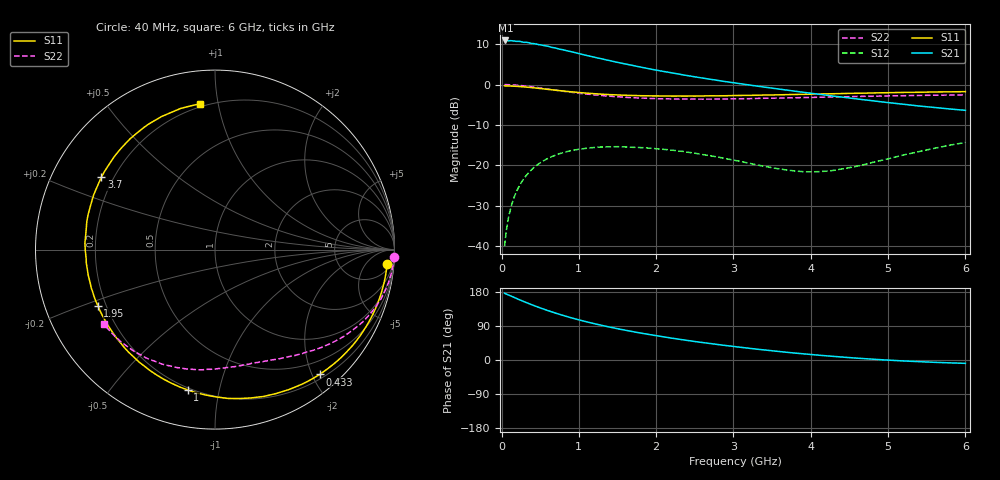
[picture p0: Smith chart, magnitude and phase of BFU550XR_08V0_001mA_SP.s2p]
! Filename:  P:\Prog\Test\Noise\ATS_data\Testdata_Net\03 Spar\BFU550XR_APG2013_45_C05_08p0V_001mA_SP_CM01_D.s2p
! Date/Time: Tue 06/Aug/2013 14:38:16
! BFU550XR_APG2013_45_C05_08p0V_1to35mA_SP_CM01_Bias1_R.s2p
! MDIF S-parameter v. bias file
! BFU550XR_APG2013_45_C05_08p0V_1to35mA_SP_CM01
! Date/time Fri Aug 02 14:53:20 2013
! bias mode 1
! bias variable = I_out
! VAR bias_var= 1
! VAR V_out= 8.0000
! VAR I_out= 0.9950
! VAR V_in= 0.7748
! VAR I_in= 0.0103
! Device data file deembeded for feedlines and parallel
! Original file: \03 Spar\BFU550XR_APG2013_45_C05_08p0V_001mA_SP_CM01_R.s2p
! Feed-files: PR006V01_02082013_Feed1.s2p, PR006V01_02082013_Feed2.s2p
! Parallel-file: PR006V01_02082013_Par.s2p
# MHz S MA R 50
!  Freq-MHz  S11-mag  S11-arg  S21-mag  S21-arg  S12-mag  S12-arg  S22-mag  S22-arg
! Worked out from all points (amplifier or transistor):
!   98 points, 40 MHz to 6 GHz, reference 50 ohm
!   highest |S21| = 10.9 dB at 50 MHz (marker M1)
!   |S21| within 3 dB of that: start of sweep to 952 MHz
!   unconditionally stable (mu >= 1): 3.435 GHz to 4.766 GHz
!   at 300 MHz: K = 0.08, MSG = 16.7 dB, |S12| = -23.0 dB
!   at 1.6 GHz: K = 0.38, MSG = 10.3 dB, |S12| = -15.4 dB
!   at 6 GHz: K = 0.77, MSG = 4.0 dB, |S12| = -14.3 dB
!   S11 on the Smith chart (normalised r, x): 40 MHz: 9, -20; 433 MHz: 0.27, -2.12; 1 GHz: 0.19, -0.81; 1.95 GHz: 0.17, -0.22; 3.7 GHz: 0.15, +0.29; 6 GHz: 0.18, +0.89
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40  0.9628 -4.8  3.503 176.4  0.01007 86.7  0.9983 -2.2
50  0.9618 -6.0  3.504 174.8  0.01249 86.2  0.997 -2.9
100  0.9592 -12.0  3.469 170.8  0.025 82.1  0.9935 -6.0
180  0.9514 -21.5  3.427 163.6  0.04437 76.0  0.9841 -10.8
320  0.929 -37.8  3.329 151.6  0.0752 65.9  0.9548 -18.6
433  0.9078 -50.0  3.181 142.6  0.09682 58.5  0.9258 -24.3
600  0.8709 -67.2  2.974 130.4  0.1222 48.3  0.8779 -31.9
700  0.8503 -76.4  2.824 123.7  0.1343 42.9  0.851 -36.0
850  0.8215 -89.3  2.608 114.4  0.1487 35.8  0.814 -41.2
1000  0.7966 -101.0  2.414 106.0  0.1587 29.3  0.7816 -46.0
1050  0.7899 -104.6  2.35 103.3  0.1608 27.3  0.7697 -47.6
1250  0.7654 -118.0  2.122 93.5  0.1687 20.1  0.7395 -52.9
1500  0.7438 -132.7  1.88 82.6  0.1707 12.4  0.7068 -59.3
1700  0.7318 -143.0  1.718 74.8  0.1675 7.3  0.685 -64.0
1950  0.7235 -154.5  1.538 65.9  0.1631 1.7  0.6728 -69.2
2050  0.7228 -158.7  1.477 62.7  0.1594 -0.0  0.667 -71.4
2500  0.7196 -176.0  1.245 48.8  0.1417 -6.8  0.6611 -80.5
3100  0.7335 164.4  1.02 33.4  0.1117 -8.0  0.6675 -92.3
3700  0.7507 147.5  0.8514 20.1  0.08771 3.0  0.6844 -103.9
4100  0.7638 137.2  0.7599 12.7  0.08392 18.0  0.6957 -111.5
5200  0.799 111.9  0.5707 -2.5  0.1349 43.2  0.7277 -131.8
6000  0.817 95.8  0.48 -8.8  0.1925 41.6  0.7457 -146.1
